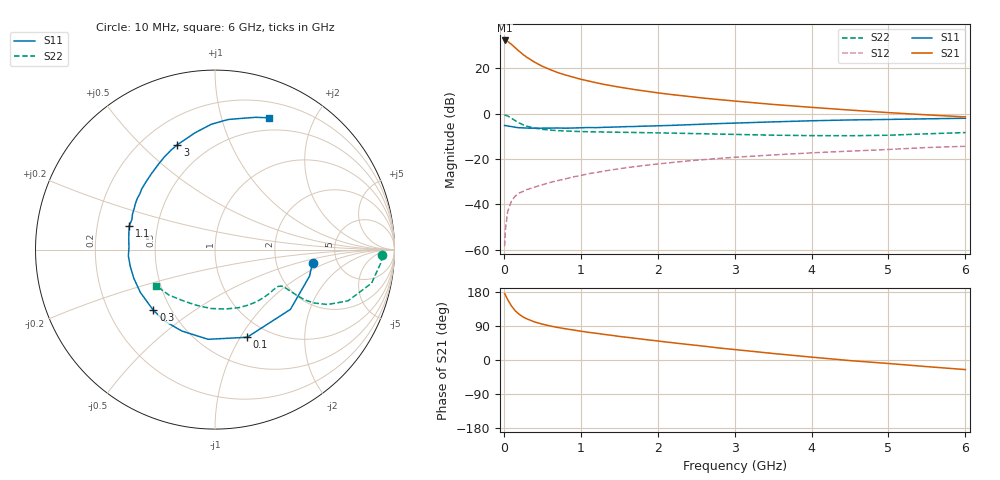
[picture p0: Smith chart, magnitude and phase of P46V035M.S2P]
! SIEMENS Small Signal Semiconductors
! BFP182
! Si NPN RF Bipolar Junction Transistor in SOT143
! VCE = 6 V  IC = 35 mA
! Common Emitter S-Parameters:  March  1996
# GHz  S  MA  R  50
!  f  S11  S21  S12  S22
! GHz  MAG  ANG  MAG  ANG  MAG  ANG  MAG  ANG
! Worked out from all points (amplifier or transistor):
!   36 points, 10 MHz to 6 GHz, reference 50 ohm
!   highest |S21| = 32.3 dB at 10 MHz (marker M1)
!   |S21| within 3 dB of that: start of sweep to 140.8 MHz
!   unconditionally stable (mu >= 1): start of sweep to 10.13 MHz; 553.3 MHz to 5.703 GHz
!   at 250 MHz: K = 0.64, MSG = 30.2 dB, |S12| = -34.2 dB
!   at 1.4 GHz: K = 1.24, MAG = 15.6 dB, |S12| = -24.8 dB
!   at 6 GHz: K = 0.97, MSG = 6.5 dB, |S12| = -14.4 dB
!   S11 on the Smith chart (normalised r, x): 10 MHz: 3.27, -0.68; 100 MHz: 0.80, -1.07; 300 MHz: 0.40, -0.35; 1.1 GHz: 0.34, +0.12; 3 GHz: 0.34, +0.65; 6 GHz: 0.36, +1.43
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0.01  0.5481 -7.6  41.19 175.2  0.0012 78.1  0.9323 -1.9
0.02  0.5471 -15.7  41.15 171.5  0.0027 79.7  0.9263 -4.7
0.05  0.5362 -38.4  39.29 159.2  0.007 81.2  0.8924 -12.1
0.1  0.5202 -69.9  33.63 142.3  0.0119 61.6  0.7938 -21.1
0.15  0.5012 -94.4  28.24 129.5  0.0154 58.1  0.6981 -26.0
0.2  0.4899 -112.2  23.76 120.5  0.0178 54.0  0.6244 -28.4
0.25  0.4871 -125.1  20.17 113.5  0.0194 52.5  0.5702 -29.3
0.3  0.4819 -135.4  17.48 108.5  0.0213 53.2  0.5306 -29.2
0.4  0.4794 -150.1  13.67 100.4  0.024 53.4  0.4808 -28.9
0.5  0.4797 -160.6  11.11 94.7  0.0271 53.8  0.4523 -28.6
0.6  0.4813 -168.8  9.42 89.9  0.0305 55.0  0.4346 -28.4
0.7  0.484 -175.8  8.066 85.9  0.0335 56.3  0.4234 -28.8
0.8  0.4795 178.5  7.147 82.4  0.0365 56.1  0.4154 -29.4
1  0.4894 168.6  5.751 76.0  0.0433 57.6  0.404 -31.1
1.1  0.4956 164.3  5.259 73.0  0.0476 57.1  0.4004 -32.3
1.5  0.5119 150.2  3.858 62.3  0.061 56.6  0.39 -37.8
2.2  0.5539 129.0  2.62 45.4  0.0844 51.6  0.3729 -50.3
3  0.6206 109.7  1.901 27.6  0.1095 44.7  0.3497 -67.8
3.5  0.6599 99.8  1.6 17.2  0.1232 40.1  0.3359 -80.3
4.5  0.7283 84.3  1.202 -1.6  0.1497 31.3  0.3268 -108.1
5.5  0.7711 72.9  0.943 -17.5  0.1794 23.1  0.3604 -135.3
6  0.7937 67.7  0.849 -25.3  0.191 18.1  0.3838 -148.2
